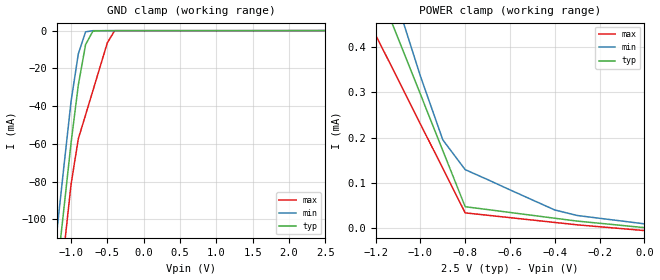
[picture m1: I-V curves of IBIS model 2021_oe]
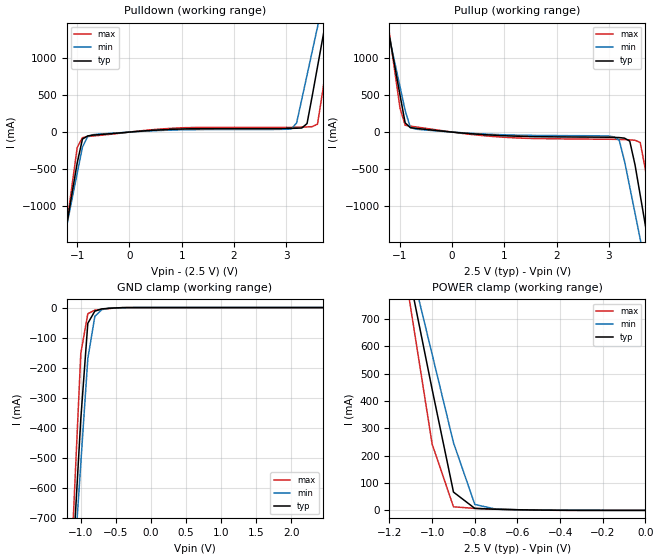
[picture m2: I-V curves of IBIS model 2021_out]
| IBIS File EG2021CA.ibs
[IBIS ver]   3.2
[File name]   eg2021ca.ibs
[File Rev]   1.0
[Date]   Aug 11,2003
[Source]   Circiuts Simulation for EG-2021CA by HSPICE
[Disclaimer] This ionformation is for modeling only,and is not guaranteed.
[Component]   EG-2021CA
[Manufacturer]   Seiko Epson Corp.
[Package]
| variable   typ   min   max
R_pkg   0.30   0.07   0.46
L_pkg   7.80nH   5.82nH   13.65nH
C_pkg   1.35pF   1.20pF   2.57pF
[Pin]   signal_name   model_name   R_pin   L_pin   C_pin
1   oe   2021_oe   0.44   5.82nH   1.35pF
2   vss   GND   0.07   7.80nH   NA
3   out   2021_out   0.44   5.82nH   1.35pF
4   vdd   POWER   0.30   13.65nH   2.57pF
| Models and submodels in the file (2): 2021_oe (Input), 2021_out (3-state)
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|   Model 2021_oe
[Model]   2021_oe
Model_type   Input
C_comp   4.50pF   3.50pF   5.50pF
Vinl = 0.75V | VIL = VCC * 0.3
Vinh = 1.75V | VIH = VCC * 0.7
|   typ   min   max
[Temperature Range]   25.00   -40.00   85.00
[Voltage Range]   2.50V   2.35V   2.65V
[POWER Clamp Reference]   2.50V   2.35V   2.65V
[GND Clamp Reference]   0.00V   0.00V   0.00V
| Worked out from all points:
|   GND clamp passes 1 mA (typ) near -0.71 V on its own axis
|   POWER clamp passes 1 mA (typ) near -1.50 V on its own axis
[GND_clamp]
|voltage   current   current   current
|vout   I(typ)   I(min)   I(max)
-2.5V     -614mA     -592mA     -635mA
-1.2V     -130mA     -108mA     -152mA
-1.1V     -94.8mA    -72.5mA    -117mA
-1V       -59.5mA    -37.5mA    -81.4mA
-900mV    -28.8mA    -12.3mA    -57.3mA
-800mV    -7.42mA    -656uA     -44.6mA
-700mV    -316uA     -41.8uA    -31.9mA
-500mV    -41.3uA    -40.2uA    -6.41mA
-400mV    -41.1uA    -40.2uA    -46.2uA
2.5V      758nA      9.12uA     -5.77uA
[POWER_clamp]
| voltage = vcc - voutput
|vout   I(typ)   I(min)   I(max)
-2.5V     2.66mA     2.82mA     2.49mA
-1.3V     669uA      819uA      525uA
-1.2V     544uA      655uA      427uA
-1.1V     420uA      492uA      329uA
-1V       296uA      336uA      230uA
-900mV    171uA      195uA      132uA
-800mV    47uA       129uA      33.4uA
-400mV    21.5uA     39.8uA     12.2uA
-300mV    15.2uA     27.6uA     6.94uA
0V        758nA      9.12uA     -5.77uA
|   Model 2021_out
[Model]   2021_out
Model_type   3-state
Polarity   Non-Inverting
Enable   Active-High
C_comp   2.50pF   1.50pF   3.50pF
Rref  = 100k  | Note: Probe Real Impedance
Cref  = 15.0pF
Vref  = 1.25V | Vref = VDD / 2
|   typ   min   max
[Temperature Range]   25.00   -40.00   85.00
[Voltage Range]   2.50V   2.35V   2.65V
[POWER Clamp Reference]   2.50V   2.35V   2.65V
[Pullup Reference]   2.50V   2.35V   2.65V
[Pulldown Reference]   2.50V   2.35V   2.65V
[GND Clamp Reference]   0.00V   0.00V   0.00V
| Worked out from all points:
|   slope of the pulldown table from 0 to 0.3 V, typ, clamps not added: 17.6 ohm
|   slope of the pullup table from 0 to 0.3 V, typ, clamps not added: 16 ohm
|   GND clamp passes 1 mA (typ) near -0.49 V on its own axis
|   POWER clamp passes 1 mA (typ) near -0.49 V on its own axis
[GND_clamp]
| voltage = voutput
| vout   I(typ)   I(min)   I(max)
-2.5V     -6.606A    -5.829A    -7.901A
-1.2V     -1.197A    -1.222A    -1.18A
-1.1V     -783.1mA   -870.2mA   -665.2mA
-1V       -370.6mA   -519.1mA   -152.4mA
-900mV    -52.33mA   -170.1mA   -20.34mA
-800mV    -11.9mA    -29.23mA   -8.762mA
-700mV    -4.442mA   -6.896mA   -5.751mA
-600mV    -2.433mA   -2.152mA   -3.302mA
-300mV    -25.05uA   -33.28uA   -14.23uA
2.5V      510.7pA    3.363uA    17.39pA
[POWER_clamp]
| voltage = vcc - voutput
|vout   I(typ)   I(min)   I(max)
-2.5V     6.286A     5.442A     7.693A
-1.2V     1.22A      1.219A     1.234A
-1.1V     831.1mA    894.8mA    737.9mA
-1V       442.8mA    571.2mA    242.5mA
-900mV    66.91mA    247.8mA    13.02mA
-800mV    7.233mA    21.57mA    7.175mA
-700mV    3.996mA    4.286mA    4.374mA
-400mV    293.7uA    487.9uA    93.5uA
0V        510.7pA    4.59nA     20.01pA
[Pullup]
| vout = vcc - voutput
|vout   I(typ)   I(min)   I(max)
-2.5V     6.398A     5.535A     7.839A
-1.3V     1.684A     1.602A     1.831A
-1.2V     1.291A     1.274A     1.33A
-1V       505.2mA    619.5mA    327.8mA
-800mV    60.11mA    61.89mA    80.61mA
3.1V      -72.09mA   -65.15mA   -97.77mA
3.2V      -74.41mA   -113.3mA   -99.72mA
3.4V      -122.9mA   -745.9mA   -105.3mA
3.6V      -854.2mA   -1.451A    -140.8mA
3.7V      -1.268A    -1.804A    -507.7mA
3.9V      -2.099A    -2.512A    -1.538A
5V        -6.681A    -6.416A    -7.229A
[Pulldown]
| voltage = voutput
|vout   I(typ)   I(min)   I(max)
-2.5V     -6.663A    -5.877A    -7.97A
-1.3V     -1.661A    -1.615A    -1.757A
-1.2V     -1.244A    -1.26A     -1.239A
-1V       -414mA     -553.6mA   -207.1mA
-800mV    -51.58mA   -60.2mA    -59.75mA
3.1V      50.31mA    43.12mA    64.31mA
3.2V      52.07mA    123.6mA    65.43mA
3.4V      115.1mA    768.6mA    69.91mA
3.6V      879.4mA    1.416A     107.4mA
3.7V      1.268A     1.74A      554.7mA
3.9V      2.046A     2.389A     1.546A
5V        6.34A      5.97A      7.02A
[Ramp]
| variable   typ   min   max
dV/dt_r   1.50/0.96n   1.41/1.10n  1.59/0.60n
dV/dt_f   1.50/0.84n   1.41/1.01n  1.59/0.65n
R_load = 100e+3
| End [Model] 2021_out
